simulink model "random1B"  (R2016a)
settings: Solver=VariableStepDiscrete  StartTime=0.0  StopTime=1e6  RelTol=1e-3
undefined symbols (not defined in the file or in its folder): Newton, Raphson

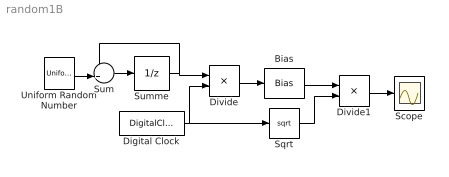
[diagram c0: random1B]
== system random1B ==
  Bias : Bias  Bias=-0.5
  Digital Clock : DigitalClock
  Divide : Product  Inputs=*/
  Divide1 : Product
  Scope : Scope
  Sqrt : Sqrt  AlgorithmType=Newton-Raphson
  Sum : Sum  Inputs=++|
  Summe : UnitDelay  SampleTime=-1
  Uniform Random Number : UniformRandomNumber  Minimum=0  SampleTime=1
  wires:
  Sum/1 -> Summe/1
  Summe/1 -> Sum/1, Divide/1
  Uniform Random Number/1 -> Sum/2
  Digital Clock/1 -> Divide/2, Sqrt/1
  Divide/1 -> Bias/1
  Bias/1 -> Divide1/1
  Sqrt/1 -> Divide1/2
  Divide1/1 -> Scope/1
